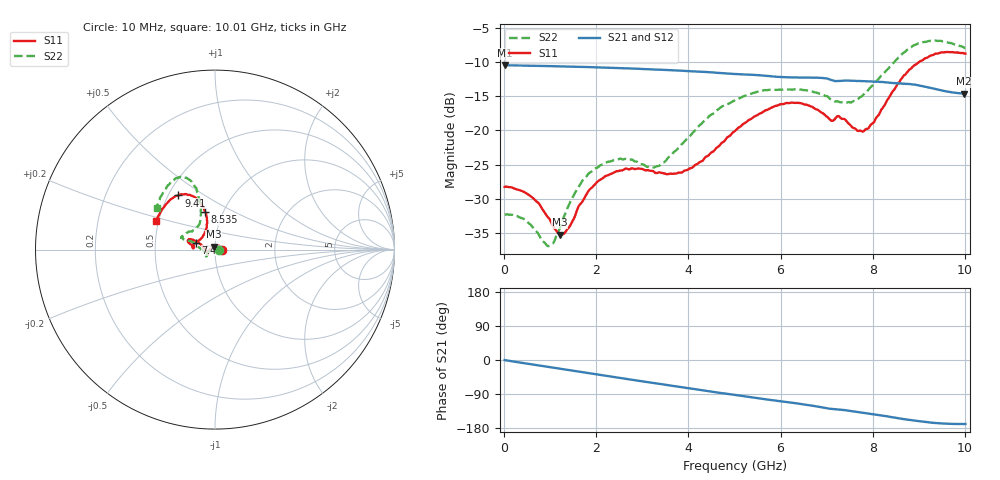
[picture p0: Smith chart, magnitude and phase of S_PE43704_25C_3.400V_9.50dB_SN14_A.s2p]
! Device ID: PE43704
! Dir: z:\PE43704\PE43704_Char_1_20130516\PE43704\AMB\3p400V\9p50dB
! Serial: 14
! Insertion: A
! Impedance: 50 ohm
! Temp: Amb
! VDD: 3.400V
! Attenuation Step: 9.50dB
! IDD: 1.140024e-01mA
#  Hz  S  RI  R  50
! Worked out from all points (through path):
!   401 points, 10 MHz to 10.01 GHz, reference 50 ohm
!   highest |S21| = -10.49 dB at 10 MHz (marker M1); lowest = -14.6 dB at 9.985 GHz (marker M2)
!   group delay of S21, straight-line fit = 48.6 ps
!   lowest |S11| = -35.2 dB at 1.21 GHz (marker M3), VSWR 1.04, Z = 49.3 + j1.59 ohm
!   |S11| at or under -10 dB: start of sweep to 9.01 GHz
!   |S22| runs from -36.9 to -6.9 dB; largest |S21 - S12| = 0.0023
!   S11 on the Smith chart (normalised r, x): 10 MHz: 1.08, +0.00; 7.46 GHz: 0.81, +0.06; 8.535 GHz: 0.82, +0.36; 9.41 GHz: 0.56, +0.39; 10.01 GHz: 0.49, +0.18
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1e7  0.0387 0.000296  0.2989 -0.00106  0.299 -0.00112  0.0242 0.00027
5.35e8  0.028 0.019  0.2917 -0.0533  0.2917 -0.0532  0.0145 0.0152
9.6e8  0.00779 0.0217  0.2796 -0.0928  0.2796 -0.0928  -0.00454 0.0136
1.21e9  -0.00638 0.0162  0.2698 -0.1152  0.2699 -0.1152  -0.0185 0.00594
1.385e9  -0.0164 0.0103  0.2619 -0.1301  0.2619 -0.13  -0.0276 -0.0013
1.685e9  -0.0298 -0.00188  0.2465 -0.1542  0.2464 -0.1541  -0.0393 -0.0158
2.01e9  -0.0392 -0.0143  0.227 -0.1778  0.2272 -0.1776  -0.0448 -0.0289
2.41e9  -0.043 -0.0252  0.2003 -0.2035  0.2004 -0.2034  -0.0486 -0.0365
3.36e9  -0.0426 -0.0252  0.1266 -0.2468  0.1268 -0.2466  -0.0525 -0.0169
4.035e9  -0.0529 -0.00235  0.0696 -0.2611  0.07 -0.2611  -0.0902 0.0132
5.01e9  -0.0915 0.0377  -0.00964 -0.2577  -0.00969 -0.2579  -0.1582 0.0503
5.96e9  -0.1419 0.0582  -0.0764 -0.2337  -0.0756 -0.2339  -0.1867 0.0663
6.685e9  -0.1444 0.0355  -0.1235 -0.2089  -0.1235 -0.2087  -0.1737 0.0824
7.085e9  -0.1175 0.0169  -0.1467 -0.1824  -0.1476 -0.183  -0.1355 0.101
7.46e9  -0.1066 0.0387  -0.1592 -0.1673  -0.1588 -0.1675  -0.1019 0.1239
7.835e9  -0.067 0.0759  -0.1749 -0.1467  -0.175 -0.147  -0.081 0.1699
8.36e9  -0.0452 0.1692  -0.1923 -0.1125  -0.1917 -0.1134  -0.0854 0.2755
8.535e9  -0.0552 0.2105  -0.1971 -0.0993  -0.1956 -0.1008  -0.0993 0.3193
8.935e9  -0.1025 0.2847  -0.2028 -0.0718  -0.2018 -0.0697  -0.1508 0.394
9.41e9  -0.2034 0.3016  -0.1937 -0.046  -0.1933 -0.045  -0.2297 0.3866
9.985e9  -0.3213 0.1703  -0.1821 -0.0361  -0.1829 -0.036  -0.3224 0.2372
1.001e10  -0.3262 0.1603  -0.1826 -0.0363  -0.1843 -0.0369  -0.3252 0.2291
